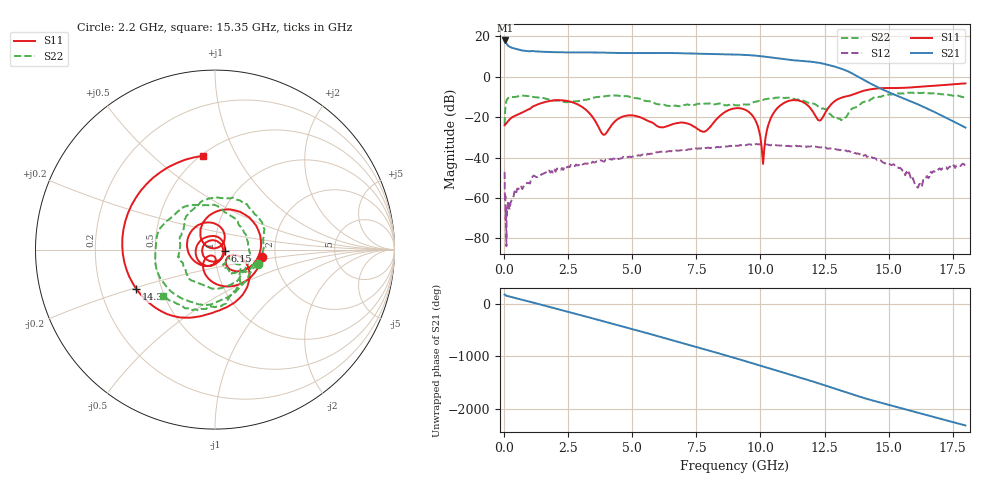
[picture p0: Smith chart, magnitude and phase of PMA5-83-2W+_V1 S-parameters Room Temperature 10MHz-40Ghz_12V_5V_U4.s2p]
!Mini-Circuits Laboratory
!S-Parameters
!Model: US-AMP-1
!Run / Lot / Date Code: N/A /  / N/A
!Fixture: ON TB-
!Network Analyzer: NFA N8975A;  Serial number: 74408
!Date: 12/1/2023 at 8:05:33 AM
!No.: Unit# 2 (#4)
!Tested with:
!Condition 2: Vdd = +12V; Vg2= +5V; Idd= 400mA
# Hz  S  dB  R  50
!Frequency  S11 dB  S11 Deg  S21 dB  S21 Deg  S12 dB  S12 Deg  S22 dB  S22 Deg
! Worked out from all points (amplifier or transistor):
!   368 points, 10 MHz to 18 GHz, reference 50 ohm
!   highest |S21| = 18.0 dB at 20 MHz (marker M1)
!   |S21| within 3 dB of that: start of sweep to 187 MHz
!   unconditionally stable (mu >= 1): start of sweep to end of sweep
!   at 2.7 GHz: K = 17.50, MAG = 12.6 dB, |S12| = -44.0 dB
!   at 8.85 GHz: K = 6.80, MAG = 11.4 dB, |S12| = -34.3 dB
!   at 18 GHz: K = 693.68, MAG = -22.0 dB, |S12| = -44.1 dB
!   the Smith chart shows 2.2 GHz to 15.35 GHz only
!   S11 on the Smith chart (normalised r, x): 2.2 GHz: 1.69, -0.15; 6.15 GHz: 1.12, -0.01; 14.3 GHz: 0.36, -0.21; 15.35 GHz: 0.51, +0.74
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1e7  -24.01 -0.0  17.83 177.4  -47.08 -7.6  -23.53 -65.0
2e7  -23.67 -3.3  18.01 173.9  -58.90 -175.6  -20.00 -93.3
5e8  -18.86 -146.1  13.66 101.5  -55.38 61.2  -9.76 138.1
1.15e9  -14.49 113.8  12.68 21.0  -48.94 -48.2  -10.04 64.7
2.2e9  -11.61 -9.3  12.14 -113.4  -46.08 -171.7  -11.99 -18.2
3.05e9  -15.05 -96.9  12.11 136.2  -43.46 83.9  -11.63 -63.9
4e9  -27.49 -91.1  11.94 10.7  -41.30 -41.1  -9.49 -132.4
4.8e9  -19.18 -139.5  11.77 -94.4  -39.83 -139.5  -9.60 161.3
5.45e9  -20.85 138.4  11.80 179.5  -38.66 134.8  -11.76 108.3
6.05e9  -24.92 17.9  11.84 98.5  -37.28 59.3  -13.67 62.7
6.15e9  -25.04 -5.7  11.83 84.8  -37.16 47.0  -13.70 55.9
6.75e9  -22.93 -124.1  11.72 2.7  -36.61 -30.9  -14.57 17.6
7.4e9  -24.67 122.6  11.50 -86.4  -35.81 -114.1  -14.00 -39.3
8.15e9  -23.00 -74.2  11.31 170.1  -35.29 143.7  -13.63 -108.2
9.05e9  -15.57 144.9  11.03 42.9  -34.22 22.2  -14.15 178.7
9.85e9  -22.94 43.7  10.43 -73.7  -33.34 -87.9  -12.18 130.7
1.055e10  -17.19 125.9  9.34 -176.1  -33.76 174.8  -10.55 73.9
1.205e10  -17.33 -53.1  7.37 -37.0  -34.48 -37.1  -13.23 -33.3
1.43e10  -6.19 -153.3  -3.36 -27.1  -39.71 -28.8  -11.23 -72.8
1.505e10  -5.54 130.8  -7.87 -126.1  -43.32 -108.3  -8.69 -117.1
1.535e10  -5.55 97.4  -9.50 -165.2  -44.85 -145.3  -8.25 -138.0
1.8e10  -3.26 160.1  -25.17 -152.6  -44.08 56.4  -10.22 46.4
